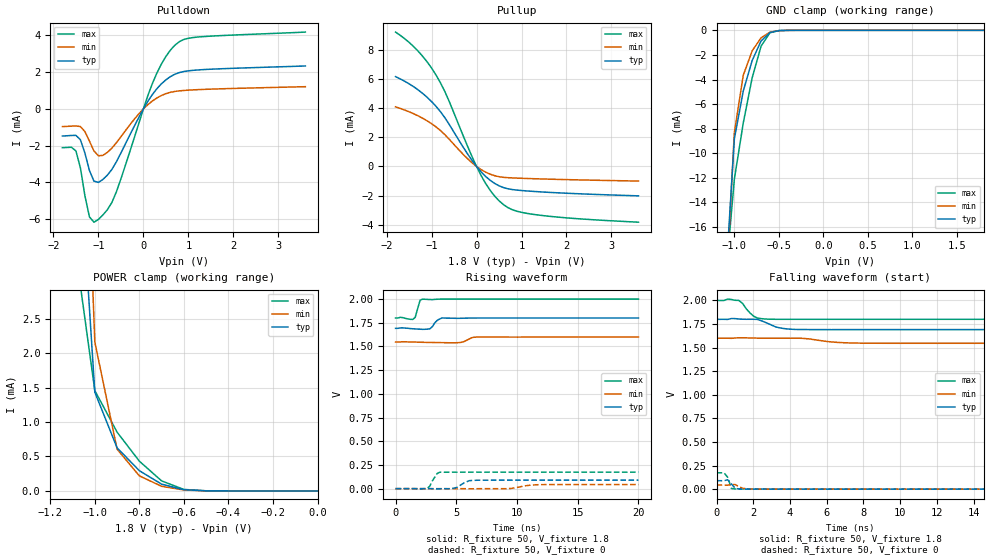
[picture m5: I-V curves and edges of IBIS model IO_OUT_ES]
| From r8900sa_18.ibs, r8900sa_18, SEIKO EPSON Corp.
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[Model]   IO_OUT_ES
Model_type 3-state
Enable Active-High
Polarity Non-Inverting
Vmeas=0.90
C_comp   2.5p   2p   3p
[Temperature Range] 25   85   -40
[Voltage Range]   1.8   1.6   2.0
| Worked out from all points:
|   slope of the pulldown table from 0 to 0.27 V, typ, clamps not added: 269 ohm
|   slope of the pullup table from 0 to 0.27 V, typ, clamps not added: 313 ohm
|   GND clamp passes 1 mA (typ) near -0.71 V on its own axis
|   POWER clamp passes 1 mA (typ) near -0.95 V on its own axis
|   falling waveform, R_fixture 50, V_fixture 1.8: 20-80 % time 843ps typ, 1.33ns min, 530ps max; typ from 1.8 V to 1.69 V
|   falling waveform, R_fixture 50, V_fixture 0: 20-80 % time 239ps typ, NA min, 211ps max; typ from 0.09 V to 0 V
|   rising waveform, R_fixture 50, V_fixture 1.8: 20-80 % time 420ps typ, 506ps min, 267ps max; typ from 1.69 V to 1.8 V
|   rising waveform, R_fixture 50, V_fixture 0: 20-80 % time 724ps typ, NA min, 469ps max; typ from 0 V to 0.09 V
[Pullup]
-1.8V     6.156mA    4.085mA    9.207mA
-1.3V     5.251mA    3.469mA    7.906mA
-1.1V     4.743mA    3.129mA    7.176mA
-900mV    4.117mA    2.71mA     6.264mA
-700mV    3.323mA    2.166mA    5.106mA
-200mV    863.4uA    532.9uA    1.39mA
100mV     -365.3uA   -212.3uA   -614.2uA
300mV     -942.3uA   -526.8uA   -1.622mA
600mV     -1.45mA    -746.8uA   -2.618mA
900mV     -1.62mA    -799.6uA   -3.073mA
1.4V      -1.738mA   -852.6uA   -3.339mA
3.6V      -2.015mA   -1.002mA   -3.82mA
[Pulldown]
-1.8V     -1.476mA   -963.3uA   -2.11mA
-1.5V     -1.439mA   -925.2uA   -2.285mA
-1.4V     -1.679mA   -961.4uA   -3.21mA
-1.2V     -3.345mA   -1.75mA    -5.87mA
-1.1V     -3.927mA   -2.283mA   -6.161mA
-900mV    -3.837mA   -2.526mA   -5.769mA
-700mV    -3.288mA   -2.131mA   -5.085mA
200mV     783.2uA    430.4uA    1.382mA
400mV     1.363mA    727.5uA    2.439mA
700mV     1.885mA    949.8uA    3.465mA
1.2V      2.116mA    1.046mA    3.906mA
3.6V      2.334mA    1.208mA    4.177mA
[GND Clamp]
-1.8V     -168.9mA   -143.4mA   -209.1mA
-1.1V     -20.64mA   -22.12mA   -20.39mA
-1V       -8.831mA   -8.329mA   -12.11mA
-900mV    -4.941mA   -3.657mA   -7.543mA
-800mV    -2.459mA   -1.675mA   -3.865mA
-700mV    -864uA     -604.2uA   -1.29mA
-600mV    -179.4uA   -151uA     -195.7uA
-500mV    -26.95uA   -29.51uA   -18.23uA
-400mV    -3.685uA   -4.954uA   -1.653uA
1.8V      45.53pA    1.656nA    26.26pA
[POWER Clamp]
-1.8V     122.7mA    107.2mA    149.1mA
-1.1V     6.482mA    10.72mA    3.807mA
-1V       1.434mA    2.163mA    1.457mA
-900mV    625.6uA    606.7uA    853.6uA
-800mV    293.7uA    218.9uA    432uA
-700mV    98.19uA    66.89uA    145.6uA
-600mV    17.36uA    13.33uA    21.68uA
-500mV    1.719uA    1.888uA    1.298uA
0V        45.59pA    162.2pA    31.43pA
[Falling Waveform]
R_fixture=50
V_fixture=1.8
V_fixture_min=1.6
V_fixture_max=2.0
0s        1.8V       1.6V       2V
606.1ps   1.799V     1.6V       2.015V
1.212ns   1.803V     1.604V     2.001V
2.02ns    1.801V     1.601V     1.833V
2.222ns   1.799V     1.601V     1.814V
2.828ns   1.753V     1.6V       1.801V
3.434ns   1.71V      1.6V       1.8V
4.242ns   1.693V     1.6V       1.8V
7.677ns   1.691V     1.548V     1.8V
20ns      1.691V     1.546V     1.8V
[Falling Waveform]
R_fixture=50
V_fixture=0
V_fixture_min=0
V_fixture_max=0
0s        89.6mV     43.32mV    173.9mV
404ps     88.95mV    43.13mV    173.1mV
606.1ps   99.82mV    42.32mV    126.4mV
808.1ps   55.87mV    47.17mV    7.841mV
1.01ns    9.69mV     49.12mV    1.709mV
1.212ns   1.941mV    28.05mV    1.657mV
1.414ns   740.4uV    9.932mV    2.321mV
1.616ns   307.3uV    4.051mV    1.68mV
2.222ns   905.7uV    539.8uV    227.4uV
20ns      37.57uV    18.18uV    1.214uV
[Rising Waveform]
R_fixture=50
V_fixture=1.8
V_fixture_min=1.6
V_fixture_max=2.0
0s        1.691V     1.546V     1.8V
1.414ns   1.687V     1.547V     1.785V
1.616ns   1.685V     1.546V     1.806V
2.02ns    1.682V     1.545V     1.988V
2.222ns   1.681V     1.544V     1.999V
2.828ns   1.686V     1.542V     1.995V
3.838ns   1.801V     1.54V      2V
5.455ns   1.798V     1.544V     2V
6.869ns   1.8V       1.6V       2V
20ns      1.8V       1.6V       2V
[Rising Waveform]
R_fixture=50
V_fixture=0
V_fixture_min=0
V_fixture_max=0
0s        0V         0V         0V
2.626ns   -55.52uV   32.63uV    4.89mV
2.828ns   -165.1uV   28.89uV    27.76mV
3.434ns   -1.99mV    22.05uV    160.5mV
3.636ns   -1.467mV   23.55uV    173.5mV
5.051ns   13.25mV    -31.47uV   173.8mV
6.263ns   86.45mV    -1.237mV   173.9mV
9.495ns   89.58mV    2.29mV     173.9mV
11.72ns   89.59mV    41.33mV    173.9mV
20ns      89.59mV    43.29mV    173.9mV
[Ramp]
R_load=50
dV/dt_r   5.375E-2/7.089E-10   2.597E-2/1.126E-9   1.043E-1/4.674E-10
dV/dt_f   6.538E-2/8.230E-10   3.236E-2/1.318E-9   1.198E-1/5.243E-10
|[End   IO_OUT_ES
